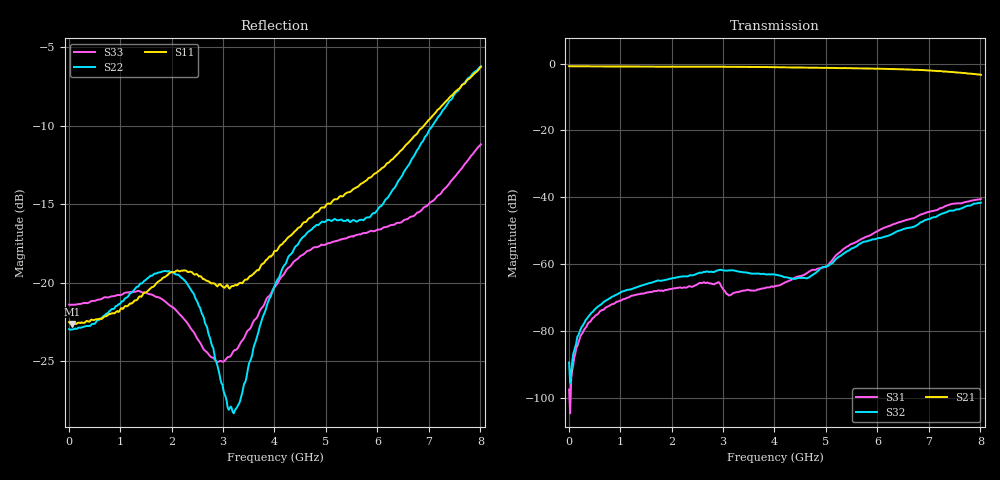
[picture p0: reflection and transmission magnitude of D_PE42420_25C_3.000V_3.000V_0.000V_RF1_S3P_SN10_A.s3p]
! Device ID: PE42420
! Serial: 10
! Insertion: A
! Temp: 25C
! VDD: 3.000
! Control_Hi: 3.000
! Control_Lo: 0.000
! Logic State: RF1
! Port 1: RFC
! Port 2: RF1
! Port 3: RF2
! V1 = 3.00
! V2 = 0.00
! V3 = 0.00
! IDD: 1.127406e-04
#  Hz  S  RI  R  50
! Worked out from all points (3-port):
!   401 points, 10 MHz to 8.01 GHz, reference 50 ohm
!   strongest paths, dB at 10 MHz, 2.01 GHz, 4.01 GHz, 6.01 GHz, 8.01 GHz:
!     S21: -0.8, -0.9, -1.1, -1.5, -3.4
!     S32: -89.5, -64.3, -63.2, -52.3, -41.6
!     S31: -97.6, -67.4, -66.7, -50.1, -40.5
!   lowest |S11| = -22.6 dB at 70 MHz (marker M1), VSWR 1.16, Z = 58 - j0.23 ohm
!   |S11| at or under -10 dB: start of sweep to 6.902 GHz
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1e7  0.0749 -0.00146  0.9087 -0.00559  -2.08e-05 -9.13e-07
     0.9121 -0.00453  0.0712 -0.00125  1.43e-06 -1.2e-05
     -8.13e-06 -1.04e-05  -3.32e-06 -3.33e-05  0.0852 -0.00106
7e7  0.0739 -0.00198  0.9067 -0.0247  -3.72e-06 2.41e-05
     0.9086 -0.0242  0.0709 -0.0024  -1.73e-06 3.09e-05
     -2.12e-06 2.53e-05  3.01e-06 3.4e-05  0.0851 -0.00384
8.1e8  0.0778 -0.0164  0.8634 -0.2556  9.36e-05 0.000216
       0.8663 -0.2549  0.0803 -0.014  0.000131 0.000283
       9.65e-05 0.000222  0.00013 0.000278  0.0812 -0.0394
1.71e9  0.098 -0.0188  0.7358 -0.5096  0.000286 0.000263
        0.7386 -0.5092  0.107 -0.00643  0.000393 0.000397
        0.000289 0.000267  0.000389 0.000397  0.0641 -0.0633
2.89e9  0.0506 -0.0832  0.4592 -0.7673  0.000497 -0.000151
        0.4616 -0.7689  0.0436 -0.0329  0.000779 0.000188
        0.000497 -0.00015  0.000774 0.00019  -0.00228 -0.0559
3.21e9  0.0125 -0.0969  0.3661 -0.8145  0.000328 -0.000169
        0.3689 -0.815  0.00103 -0.0384  0.00079 -4.83e-05
        0.000328 -0.000166  0.000796 -4.5e-05  -0.0277 -0.0541
4.01e9  -0.0865 -0.0922  0.1216 -0.8711  2.29e-05 -0.000474
        0.126 -0.8707  -0.0864 -0.0475  0.000532 -0.000411
        1.37e-05 -0.000463  0.000548 -0.000424  -0.0874 -0.0428
4.65e9  -0.1528 -0.0449  -0.0738 -0.8624  -0.000631 -0.000394
        -0.0711 -0.8641  -0.1364 -0.0495  9.91e-05 -0.000579
        -0.000652 -0.000362  0.000123 -0.000605  -0.1227 -0.0311
6.63e9  -0.1988 0.2008  -0.6191 -0.5272  -0.00402 0.00227
        -0.6185 -0.5235  -0.0998 0.2191  -0.00255 0.00249
        -0.00402 0.00241  -0.0026 0.00234  -0.1214 0.1069
8.01e9  -0.0567 0.4831  -0.6699 -0.0978  -0.0042 0.00837
        -0.6694 -0.0977  -0.0257 0.4887  -0.00241 0.00807
        -0.00419 0.00844  -0.00272 0.00782  -0.00528 0.276
